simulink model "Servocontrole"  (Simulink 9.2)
settings: Solver=ode45  StartTime=0.0  StopTime=10  MaxStep=1e-3  RelTol=1e-3  EnableMultiTasking=on
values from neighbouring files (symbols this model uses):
  A = [0 1;0 0]    [ProjetoAerogangorra.m]
  B = [0;l/J]    [ProjetoAerogangorra.m]
  C = [1 0]    [ProjetoAerogangorra.m]
  f = 1    [ProjetoAerogangorra.m]
  J = 0.1    [ProjetoAerogangorra.m]
  K = [alfa0-a0,alfa1-a1]*inv(P)    [ProjetoAerogangorra.m]
  l = 0.2    [ProjetoAerogangorra.m]
  L = Q*[alfa0-a0;alfa1-a1]    [ProjetoAerogangorra.m]
  N = -1/(C*inv(A-B*K)*B)    [ProjetoAerogangorra.m]
undefined symbols (not defined in the file or in its folder): x0

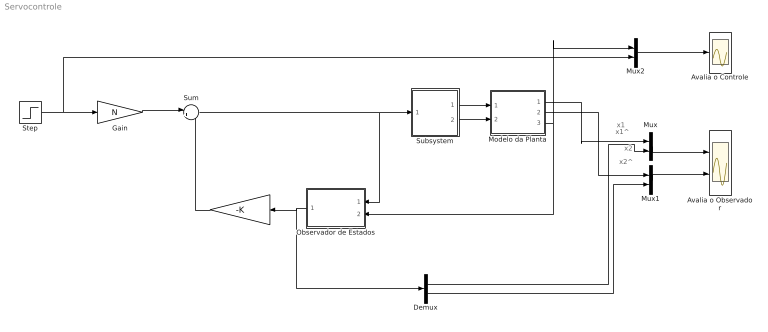
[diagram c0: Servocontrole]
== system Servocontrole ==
  note: x2^
  note: x2
  note: x1
  note: x1^
  "   " : Gain  Gain=-K  Multiplication=Matrix(K*u)
  Avalia o Controle : Scope
  Avalia o Observador : Scope  NumInputPorts=2
  Demux : Demux  Outputs=2
  Gain : Gain  Gain=N
  Modelo da Planta : Subsystem
  Mux : Mux  Inputs=2
  Mux1 : Mux  Inputs=2
  Mux2 : Mux  Inputs=2
  Observador de Estados : Subsystem
  Step : Step  SampleTime=0
  Subsystem : Subsystem
  Sum : Sum  Inputs=|++
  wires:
  Modelo da Planta/3(y) -> Mux2/1, Observador de Estados/2(y)
  Modelo da Planta/1(x1) -> Mux/1
  "   "/1 -> Sum/2
  Demux/1 -> Mux/2
  Mux/1 -> Avalia o Observador/1
  Mux1/1 -> Avalia o Observador/2
  Modelo da Planta/2(x2) -> Mux1/1
  Demux/2 -> Mux1/2
  Observador de Estados/1(x^) -> Demux/1, "   "/1
  Sum/1 -> Subsystem/1(u), Observador de Estados/1(u)
  Step/1 -> Mux2/2, Gain/1
  Gain/1 -> Sum/1
  Mux2/1 -> Avalia o Controle/1
  Subsystem/1(f1) -> Modelo da Planta/1(f1)
  Subsystem/2(f2) -> Modelo da Planta/2(f2)

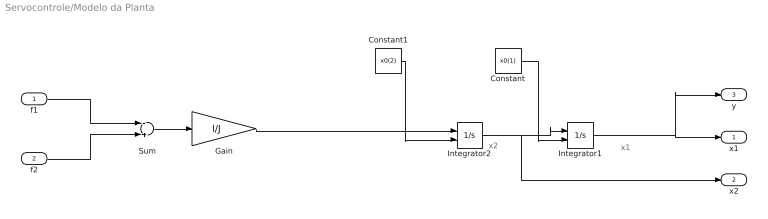
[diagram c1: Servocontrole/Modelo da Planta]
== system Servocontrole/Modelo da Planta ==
  note: x2
  note: x1
  f1 : Inport
  f2 : Inport  Port=2
  Constant : Constant  Value=x0(1)
  Constant1 : Constant  Value=x0(2)
  Gain : Gain  Gain=l/J
  Integrator1 : Integrator  InitialConditionSource=external
  Integrator2 : Integrator  InitialConditionSource=external
  Sum : Sum  Inputs=-+
  x1 : Outport
  x2 : Outport  Port=2
  y : Outport  Port=3
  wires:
  Constant/1 -> Integrator1/2
  f1/1 -> Sum/1
  f2/1 -> Sum/2
  Sum/1 -> Gain/1
  Gain/1 -> Integrator2/1
  Integrator2/1 -> x2/1, Integrator1/1
  Constant1/1 -> Integrator2/2
  Integrator1/1 -> y/1, x1/1

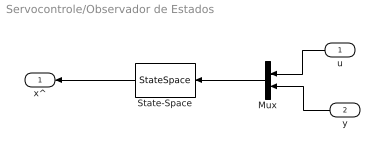
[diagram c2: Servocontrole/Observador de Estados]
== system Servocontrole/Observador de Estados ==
  u : Inport
  y : Inport  Port=2
  Mux : Mux  Inputs=2
  State-Space : StateSpace  A=A-L*C  B=[B,L]  C=eye(2)  D=zeros(2,2)  InitialCondition=x0
  x^ : Outport
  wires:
  State-Space/1 -> x^/1
  u/1 -> Mux/1
  y/1 -> Mux/2
  Mux/1 -> State-Space/1

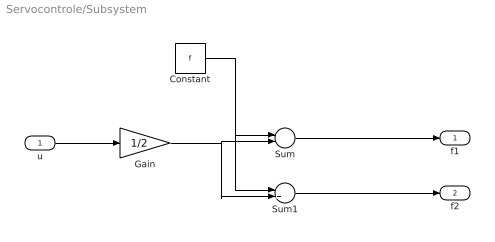
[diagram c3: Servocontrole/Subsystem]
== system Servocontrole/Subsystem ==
  u : Inport
  Constant : Constant  Value=f
  Gain : Gain  Gain=1/2
  Sum : Sum  Inputs=+-
  Sum1 : Sum
  f1 : Outport
  f2 : Outport  Port=2
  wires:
  u/1 -> Gain/1
  Sum/1 -> f1/1
  Constant/1 -> Sum1/1, Sum/1
  Gain/1 -> Sum1/2, Sum/2
  Sum1/1 -> f2/1
